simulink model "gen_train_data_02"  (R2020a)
settings: Solver=ode45  StartTime=0.0  StopTime=3000  RelTol=1e-3  EnableMultiTasking=on
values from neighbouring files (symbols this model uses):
  Ts = 0.05    [init_model.m]

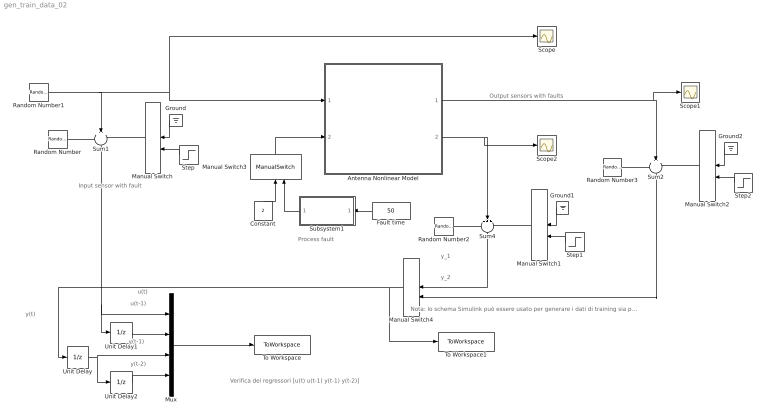
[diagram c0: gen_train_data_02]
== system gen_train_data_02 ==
  note: Nota: lo schema Simulink può essere usato per generare i dati di training sia per la prima uscita, sia per la seconda uscita, sia per le reti neurali, sia per i modelli fuzzy
  note: Verifica dei regressori [u(t) u(t-1) y(t-1) y(t-2)]
  note: y(t)
  note: y(t-1)
  note: y_2
  note: y_1
  note: u(t)
  note: Output sensors with faults
  note: Process fault
  note: Input sensor with fault
  note: u(t-1)
  note: y(t-2)
  Antenna Nonlinear Model : Subsystem
  Constant : Constant  Value=2
  Fault time : Constant  Value=50
  Ground : Ground
  Ground1 : Ground
  Ground2 : Ground
  Manual Switch{,1..4} (5 alike) : ManualSwitch
  Mux : Mux
  Random Number : RandomNumber  Variance=0.0001  Seed=1  SampleTime=Ts
  Random Number1 : RandomNumber  Variance=0.1  SampleTime=10
  Random Number2 : RandomNumber  Variance=0.00001  Seed=2  SampleTime=Ts
  Random Number3 : RandomNumber  Variance=0.00001  Seed=3  SampleTime=Ts
  Scope : Scope
  Scope1 : Scope
  Scope2 : Scope
  Step : Step  Time=50  SampleTime=0
  Step1 : Step  Time=1500  SampleTime=0
  Step2 : Step  Time=50  SampleTime=0
  Subsystem1 : Subsystem
  Sum1 : Sum  Inputs=+++  SaturateOnIntegerOverflow=on
  Sum2 : Sum  Inputs=+++  SaturateOnIntegerOverflow=on
  Sum4 : Sum  Inputs=+++  SaturateOnIntegerOverflow=on
  To Workspace : ToWorkspace  VariableName=Psim  SampleTime=Ts
  To Workspace1 : ToWorkspace  VariableName=Tsim  SampleTime=Ts
  Unit Delay : UnitDelay  SampleTime=Ts  HasFrameUpgradeWarning=on
  Unit Delay1 : UnitDelay  SampleTime=Ts  HasFrameUpgradeWarning=on
  Unit Delay2 : UnitDelay  SampleTime=Ts  HasFrameUpgradeWarning=on
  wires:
  Random Number1/1 -> Scope/1, Antenna Nonlinear Model/1(force), Sum1/2
  Random Number/1 -> Sum1/1
  Manual Switch/1 -> Sum1/3
  Sum1/1 -> Unit Delay1/1, Mux/1
  Ground/1 -> Manual Switch/1
  Step/1 -> Manual Switch/2
  Random Number2/1 -> Sum4/1
  Sum4/1 -> Manual Switch4/1
  Ground1/1 -> Manual Switch1/1
  Manual Switch1/1 -> Sum4/3
  Step1/1 -> Manual Switch1/2
  Antenna Nonlinear Model/2(velocity) -> Sum4/2, Scope2/1
  Random Number3/1 -> Sum2/1
  Ground2/1 -> Manual Switch2/1
  Manual Switch2/1 -> Sum2/3
  Step2/1 -> Manual Switch2/2
  Antenna Nonlinear Model/1(angle) -> Sum2/2, Scope1/1
  Sum2/1 -> Manual Switch4/2
  Fault time/1 -> Subsystem1/1(Fault time)
  Subsystem1/1(Fault) -> Manual Switch3/2
  Manual Switch3/1 -> Antenna Nonlinear Model/2(drag)
  Constant/1 -> Manual Switch3/1
  Mux/1 -> To Workspace/1
  Manual Switch4/1 -> To Workspace1/1, Unit Delay/1
  Unit Delay1/1 -> Mux/2
  Unit Delay/1 -> Unit Delay2/1, Mux/3
  Unit Delay2/1 -> Mux/4

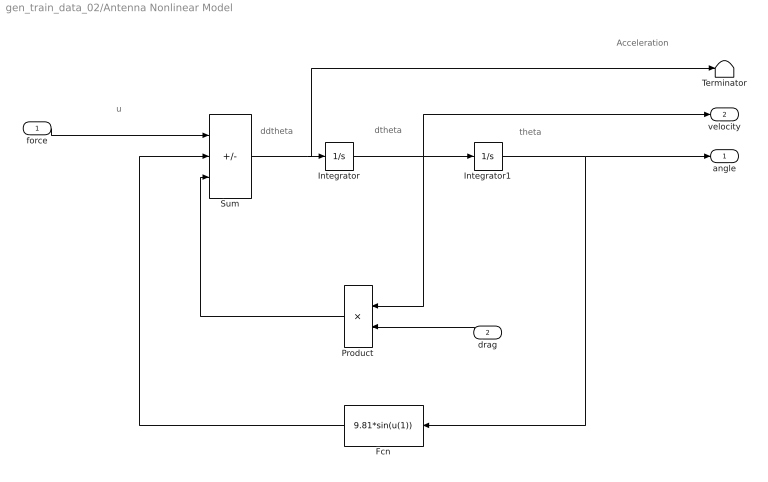
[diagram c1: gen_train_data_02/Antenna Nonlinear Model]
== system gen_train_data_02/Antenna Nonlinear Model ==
  note: Acceleration
  note: ddtheta
  note: dtheta
  note: theta
  note: u
  force : Inport
  drag : Inport  Port=2
  Fcn : Fcn  Expr=9.81*sin(u(1))
  Integrator : Integrator
  Integrator1 : Integrator  InitialCondition=(pi/180)*90
  Product : Product
  Sum : Sum  Inputs=+--  SaturateOnIntegerOverflow=on
  Terminator : Terminator
  angle : Outport
  velocity : Outport  Port=2
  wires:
  Sum/1 -> Terminator/1, Integrator/1
  Integrator/1 -> Product/1, Integrator1/1, velocity/1
  Integrator1/1 -> angle/1, Fcn/1
  Fcn/1 -> Sum/2
  Product/1 -> Sum/3
  force/1 -> Sum/1
  drag/1 -> Product/2

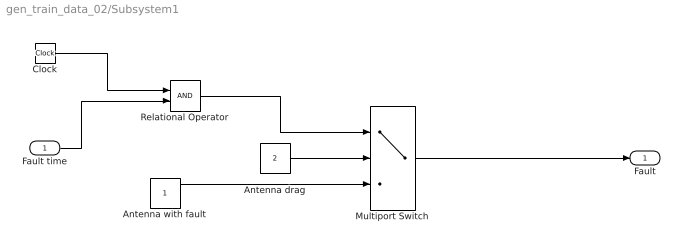
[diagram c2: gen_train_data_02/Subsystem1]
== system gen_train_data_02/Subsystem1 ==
  Fault time : Inport
  Antenna drag : Constant  Value=2
  Antenna with fault : Constant
  Clock : Clock
  Multiport Switch : MultiPortSwitch  DataPortOrder=Zero-based contiguous  Inputs=2  zeroidx=on
  Relational Operator : RelationalOperator  OutDataTypeStr=boolean  RndMeth=Simplest
  Fault : Outport
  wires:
  Clock/1 -> Relational Operator/1
  Fault time/1 -> Relational Operator/2
  Antenna drag/1 -> Multiport Switch/2
  Relational Operator/1 -> Multiport Switch/1
  Multiport Switch/1 -> Fault/1
  Antenna with fault/1 -> Multiport Switch/3
